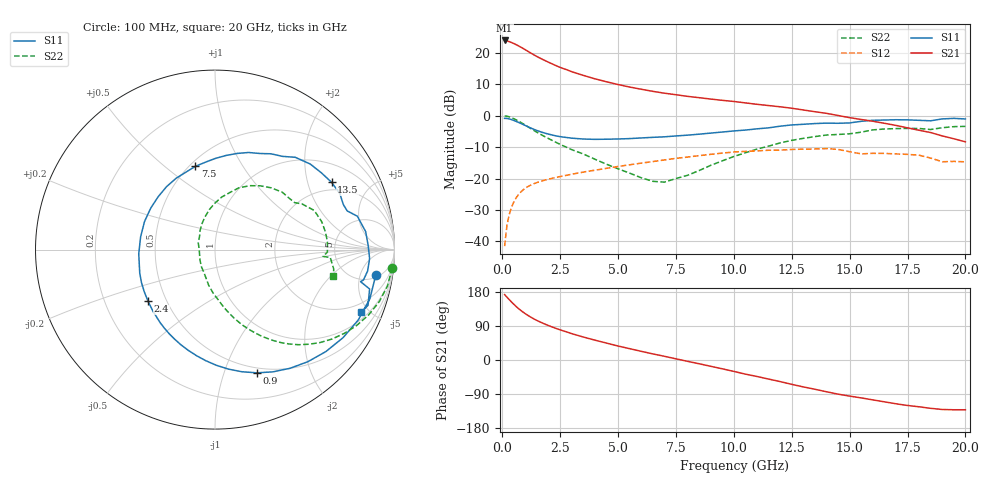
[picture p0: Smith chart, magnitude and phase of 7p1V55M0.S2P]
! Infineon Technologies  Discrete & RF Semiconductors
! bfp620
! VCE =  1.5 V,  IC =  5.0 mA
! Common Emitter S-Parameters:  Sep 2002
# GHz  S  MA  R  50
!  f  S11  S21  S12  S22
! GHz  MAG  ANG  MAG  ANG  MAG  ANG  MAG  ANG
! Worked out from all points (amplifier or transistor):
!   59 points, 100 MHz to 20 GHz, reference 50 ohm
!   highest |S21| = 23.9 dB at 100 MHz (marker M1)
!   |S21| within 3 dB of that: start of sweep to 1.003 GHz
!   unconditionally stable (mu >= 1): 4.871 GHz to 11.6 GHz; 14.79 GHz to 15.24 GHz; 17.12 GHz to end of sweep
!   at 1 GHz: K = 0.31, MSG = 22.0 dB, |S12| = -23.0 dB
!   at 5.5 GHz: K = 1.04, MAG = 11.2 dB, |S12| = -15.6 dB
!   at 20 GHz: K = 1.41, MAG = -0.6 dB, |S12| = -14.7 dB
!   S11 on the Smith chart (normalised r, x): 100 MHz: 6, -9; 900 MHz: 0.45, -1.29; 2.4 GHz: 0.40, -0.29; 7.5 GHz: 0.53, +0.64; 13.5 GHz: 1.66, +2.85; 20 GHz: 1.37, -4.49
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0.1  0.9073 -8.8  15.75 172.6  0.0084 83.0  0.9921 -5.9
0.2  0.9052 -17.6  15.5 165.9  0.0179 81.1  0.9823 -11.9
0.3  0.8892 -26.2  15.09 159.3  0.0268 76.7  0.9601 -17.6
0.4  0.866 -34.5  14.6 152.9  0.0351 72.2  0.9303 -23.0
0.5  0.8393 -42.6  14.06 146.9  0.0426 68.0  0.8959 -28.1
0.6  0.8112 -50.3  13.5 141.1  0.0495 64.1  0.8588 -32.9
0.7  0.7824 -57.7  12.91 135.8  0.0556 60.5  0.8204 -37.4
0.9  0.7248 -71.3  11.74 126.2  0.0661 54.3  0.7431 -45.2
1.2  0.6447 -89.3  10.09 114.2  0.0778 47.1  0.6347 -54.7
1.5  0.5806 -104.9  8.728 104.2  0.0865 41.8  0.5441 -62.0
1.9  0.5207 -122.8  7.373 93.2  0.0957 37.0  0.4519 -69.6
2.4  0.4712 -142.4  6.081 81.6  0.1058 32.6  0.3643 -77.3
3  0.4392 -162.7  5.01 69.5  0.1171 28.5  0.2882 -85.3
3.5  0.4255 -176.8  4.382 60.6  0.1268 25.4  0.2461 -91.9
5  0.4262 147.1  3.134 36.9  0.1556 16.2  0.143 -115.3
7  0.4612 110.4  2.282 9.8  0.1977 2.6  0.0877 179.3
7.5  0.4765 103.3  2.157 3.1  0.2099 -1.6  0.1001 158.7
10.5  0.5912 64.9  1.6 -37.3  0.2708 -30.7  0.2573 90.5
12  0.6814 49.0  1.386 -57.0  0.2832 -45.5  0.3688 68.9
13.5  0.75 30.0  1.158 -77.2  0.2956 -61.5  0.4652 47.7
17  0.8628 -3.3  0.701 -115.5  0.2467 -92.1  0.6234 8.9
20  0.8873 -23.1  0.384 -131.3  0.1846 -106.3  0.6765 -12.6
